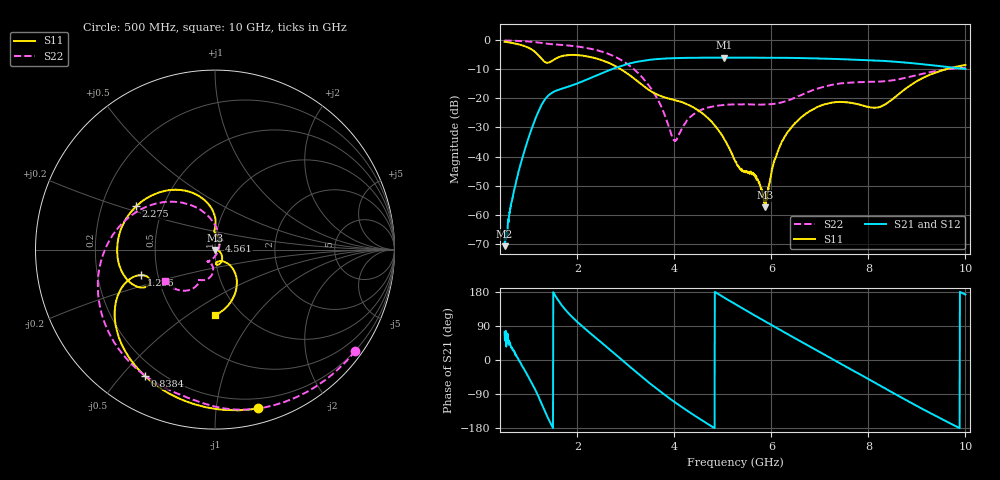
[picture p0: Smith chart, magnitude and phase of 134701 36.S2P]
!  2-Port S-parameters saved by WinCal
! VAR MeasName=S-Parameters (CALIBRATED_DATA) read from VNA (N5242A)
! VAR MeasDate=2013-7-3 16:36:45
! VAR NAME=134701 36
! VAR FILENAME=134701 36.S2P
! VAR DATE=2013-7-3 16:36:45
! VAR PHYS_PORTS=1,2
# Hz S MA R 50
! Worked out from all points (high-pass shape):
!   1601 points, 500 MHz to 10 GHz, reference 50 ohm
!   highest |S21| = -6.20 dB at 5.03 GHz (marker M1); lowest = -70.7 dB at 500 MHz (marker M2)
!   |S21| within 3 dB of the highest: 2.872 GHz to 9.533 GHz (6.661 GHz wide, 107 % of centre)
!   lowest |S11| = -57.3 dB at 5.867 GHz (marker M3), VSWR 1.00, Z = 50 - j0.132 ohm
!   |S11| at or under -10 dB: 2.882 GHz to 9.635 GHz (6.752 GHz wide, 108 % of centre)
!   |S22| runs from -34.7 to -0.3 dB; largest |S21 - S12| = 0.0018
!   S11 on the Smith chart (normalised r, x): 500 MHz: 0.12, -1.30; 838.4 MHz: 0.14, -0.58; 1.296 GHz: 0.40, -0.14; 2.275 GHz: 0.35, +0.23; 4.561 GHz: 1.04, +0.11; 10 GHz: 0.76, -0.64
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5e8  0.9175 -74.7  0.0002934 73.1  0.000339 68.7  0.9634 -35.9
8.384375e8  0.805 -119.0  0.007795 -9.6  0.007871 -10.5  0.9401 -59.9
1.064062e9  0.6711 -146.4  0.03072 -61.6  0.03071 -61.9  0.9142 -76.1
1.295625e9  0.4362 -161.0  0.08525 -124.8  0.08506 -125.0  0.8657 -92.3
1.604375e9  0.4944 -156.5  0.1378 157.6  0.1374 157.3  0.8159 -111.6
2.085312e9  0.5331 165.7  0.1894 90.4  0.1886 90.3  0.7414 -145.2
2.275312e9  0.5008 151.1  0.2202 69.6  0.2189 69.6  0.6947 -159.7
2.94625e9  0.2927 103.6  0.3628 -2.8  0.3618 -2.6  0.4245 143.4
3.670625e9  0.1123 91.0  0.4652 -79.4  0.4647 -79.4  0.08986 76.9
4.009062e9  0.0922 90.2  0.4795 -111.3  0.48 -111.3  0.01862 -19.0
4.56125e9  0.05624 64.9  0.4881 -158.5  0.4883 -158.5  0.06305 -112.4
5.030312e9  0.01965 25.1  0.4896 164.5  0.4893 164.5  0.07639 -120.9
5.25e9  0.008482 -15.3  0.4888 147.8  0.489 147.8  0.07809 -122.0
5.6775e9  0.004487 -124.3  0.4878 116.1  0.4887 116.1  0.07709 -118.5
5.8675e9  0.001361 -76.0  0.4873 102.3  0.4877 102.2  0.07747 -114.5
6.0575e9  0.008081 -8.7  0.4873 88.4  0.4872 88.5  0.07943 -108.4
6.235625e9  0.01896 -15.4  0.4863 75.5  0.486 75.5  0.08537 -102.7
6.835312e9  0.06219 -50.6  0.4774 32.1  0.4774 32.2  0.1343 -96.0
7.55375e9  0.0845 -82.8  0.4579 -18.7  0.458 -18.7  0.1813 -110.3
8.420625e9  0.08566 -52.7  0.4253 -80.5  0.4246 -80.5  0.1965 -117.0
9.234062e9  0.2427 -60.4  0.369 -137.4  0.3696 -137.3  0.2718 -123.5
1e10  0.3665 -90.3  0.3148 172.7  0.3152 172.7  0.3284 -148.1
